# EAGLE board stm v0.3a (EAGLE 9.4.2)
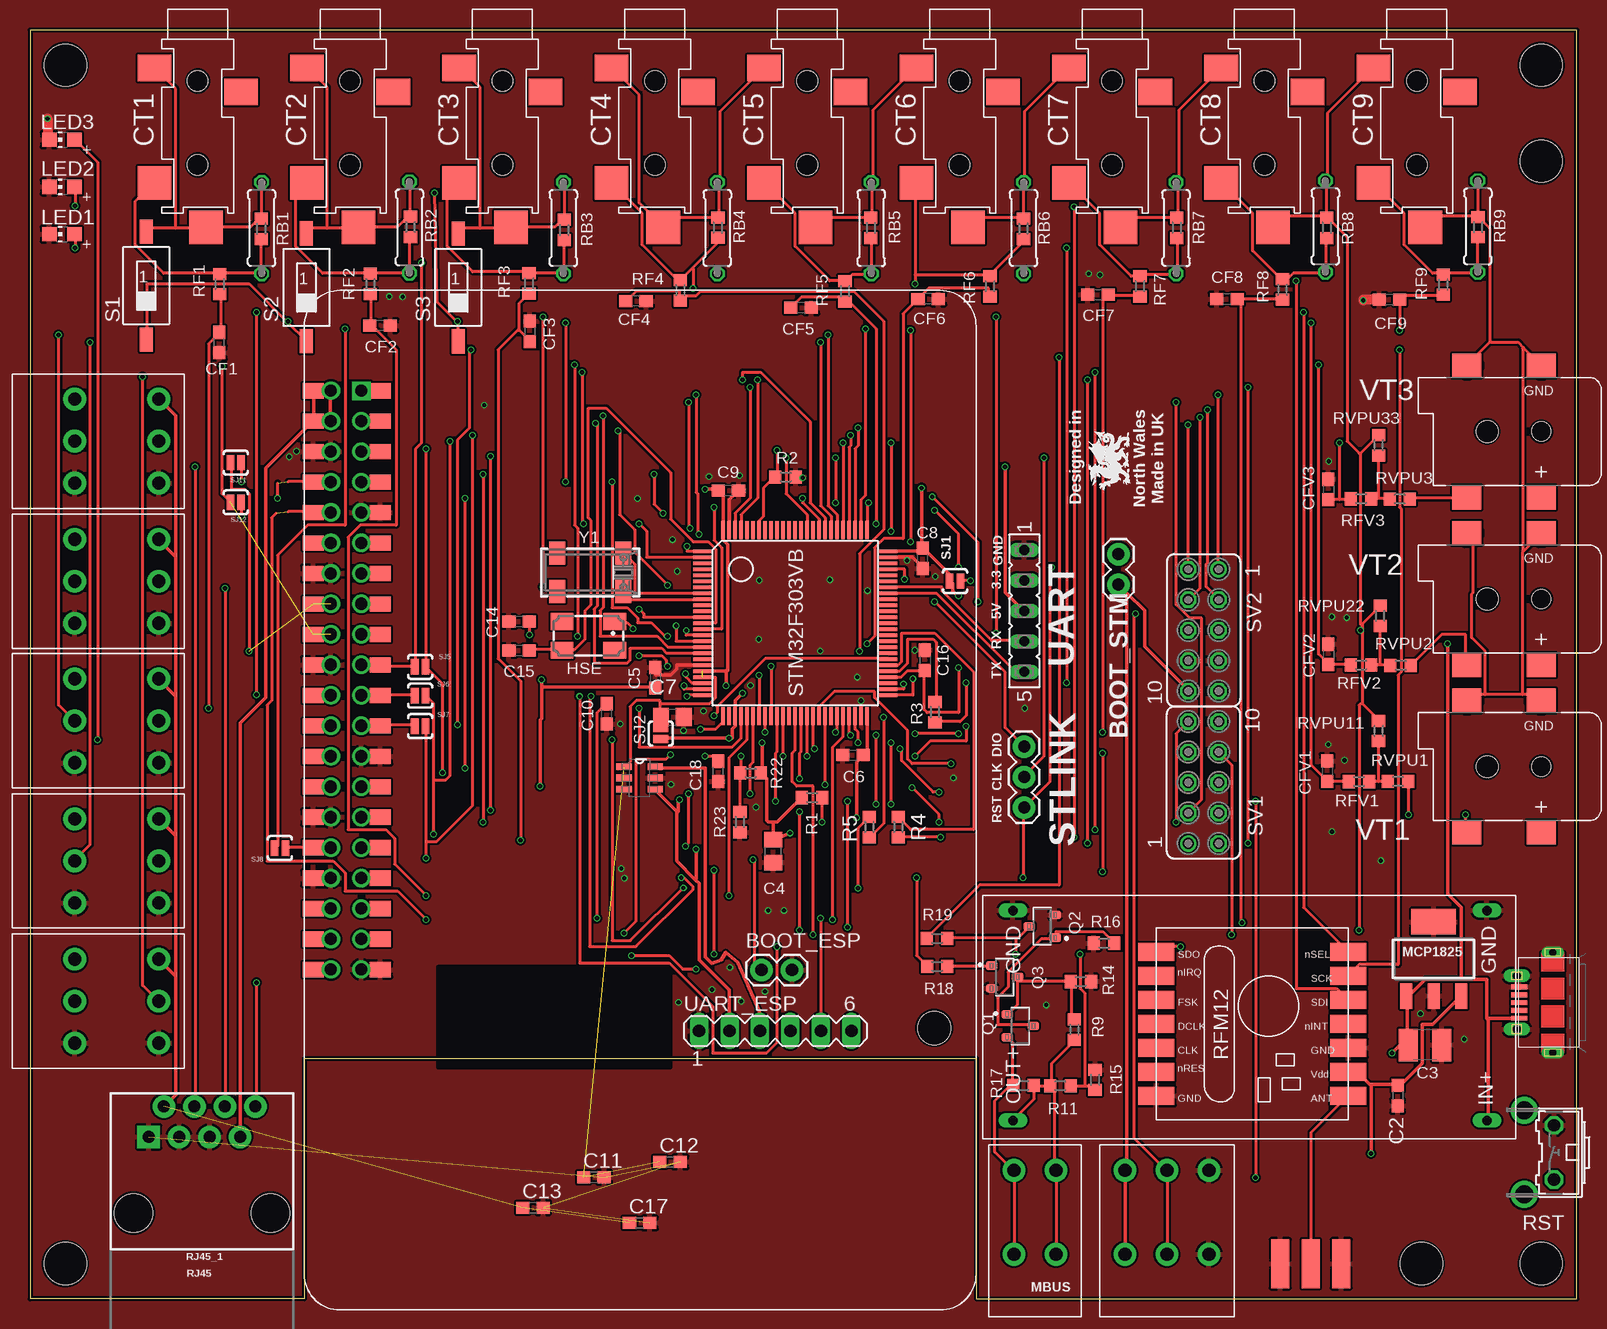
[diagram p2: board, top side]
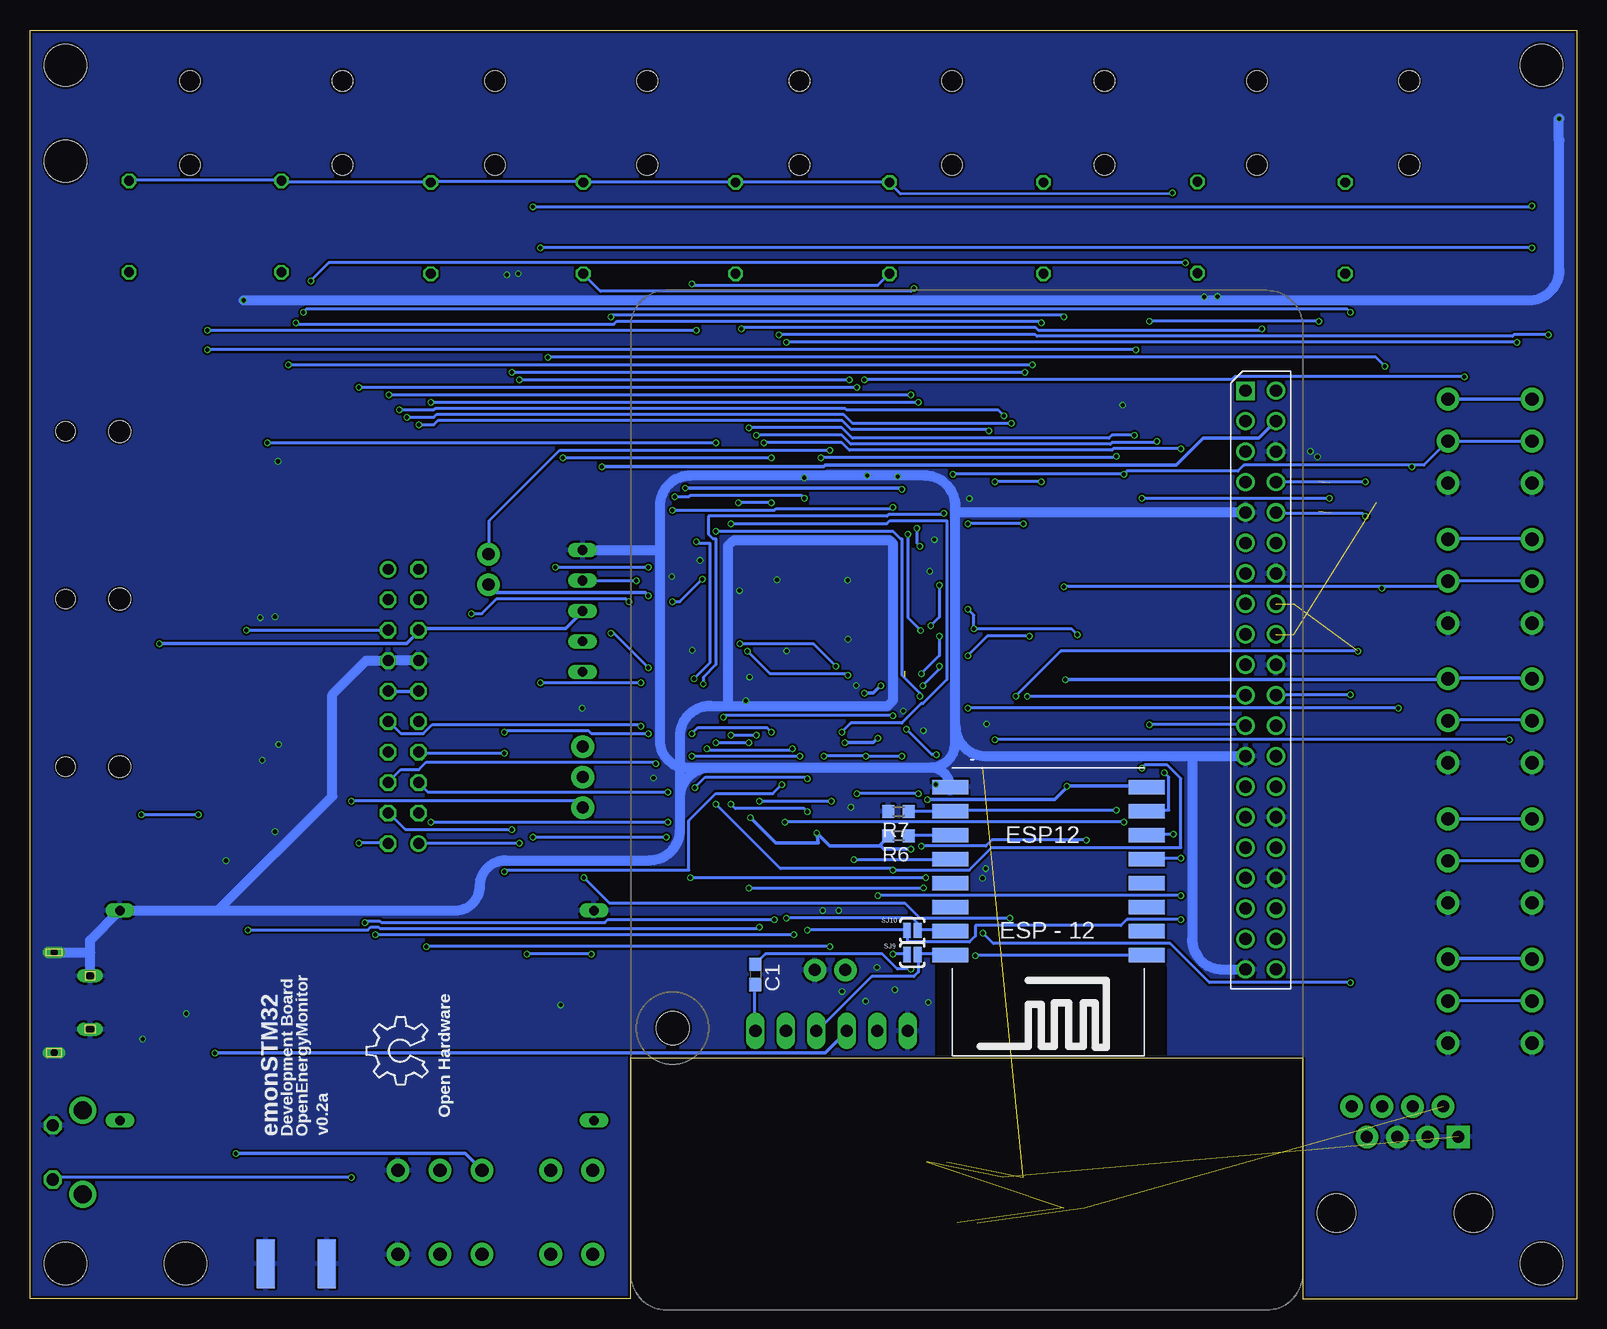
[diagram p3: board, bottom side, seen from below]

Size 128.91 x 105.79 mm. Coordinates in mm from the lower left corner, seen from the top.
Outline: 128.91,105.79 0,105.79 0,0 22.86,0 22.86,20.07 78.87,20.07 78.87,0 128.91,0 128.91,105.79
Copper layers (1*16): Top 0.035mm / dielectric 1.53mm / Bottom 0.035mm
Design rules "jlcpcb *": minimum track width 6mil, minimum drill 0.35mm, track to track 6mil, track to pad 6mil, pad to pad 7mil, via to via 8mil, smd to smd 0mil, copper to edge 8mil, drill to drill 10mil, minimum pad ring 3mil, minimum via ring 3mil, stop-mask expansion 2mil, vias tented up to drill 25mil, thermal gap 8mil
Net classes: 0 default: width 0.203 mm, drill 0.35 mm, clearance 0.152 mm; 1 power: width 0.279 mm, drill 0.35 mm, clearance 0.178 mm; 2 gnd: width 0.254 mm, drill 0.35 mm, clearance 0.152 mm
Holes 3.5 mm at 125.95,102.85 2.95,102.85 2.95,2.95 125.95,2.95 125.95,94.85 115.95,2.95
tRestrict: area 34,19.3 to 53.3,27.7
bRestrict: area 34.2,19.3 to 53.5,27.7

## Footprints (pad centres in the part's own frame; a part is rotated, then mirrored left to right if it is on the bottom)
OMNIMATE_LSF_2 = drill 1.1 pad 1.9: P$1 -3.5,-3.5; P$2 -3.5,3.5; P$3 0,-3.5; P$4 0,3.5
OMNIMATE_LSF_3 = drill 1.1 pad 1.9: P$1 -3.5,-3.5; P$2 -3.5,3.5; P$3 0,-3.5; P$4 0,3.5; P$5 3.5,-3.5; P$6 3.5,3.5
1X02 = drill 1.016 pad 1.88: 1 0,0; 2 2.54,0
C0603 = smd 1.1 x 1: 1 -0.85,0; 2 0.85,0
C1210 = smd 1.6 x 2.7: 1 -1.4,0; 2 1.4,0
C0805 = smd 1.3 x 1.5: 1 -0.95,0; 2 0.95,0
STEREO_SMT = smd 2.8 x 2.2: P$1 -3.6,-2.4; P$3 3.6,-4.4 | smd 2.8 x 2.8: P$2 -3.6,-12; P$4 0.7,-15.7 | hole 1.7: 0,-3.5; 0,-10.5
ESP12-SMD = smd 3 x 1.2: ADC -8.3,3.8; CH_PD -8.3,1.8; GND 8.1,-8.2; GPIO0 8.1,-2.2; GPIO2 8.1,-4.2; GPIO4 8.1,-0.2; GPIO5 8.1,1.8; GPIO12 -8.3,-4.2; GPIO13 -8.3,-6.2; GPIO14 -8.3,-2.2; GPIO15 8.1,-6.2; GPIO16 -8.3,-0.2; RESET -8.3,5.8; RXD0 8.1,3.8; TXD0 8.1,5.8; VCC -8.3,-8.2
FE05-1 = drill 0.813 long: 1 -5.08,0; 2 -2.54,0; 3 0,0; 4 2.54,0; 5 5.08,0
CTS406 = smd 1.9 x 1.4: 1 -2.2,-1.2; 2 2.2,-1.2; 3 2.2,1.2; 4 -2.2,1.2
SMA-EDGE = smd 1.524 x 4.064: GND@0 0,0; GND@1 5.08,0; SIG 2.54,0 | smd 1.524 x 4.064 bottom: GND@2 0,0; GND@3 5.08,0
CHIP-LED0805 = smd 1.2 x 1.2: A 0,-1.05; C 0,1.05
SOT-223 = smd 1 x 2.1: 1 -2.3,-3.1; 2 0,-3.1; 3 2.3,-3.1 | smd 3.7 x 2.1: 4 0,3.1
RPI3MIRROR2 = drill 1.016 square: P$1 8.37,4.775 | drill 1.016: P$2 8.357,2.233; P$3 10.897,4.773; P$4 10.897,2.233; P$5 13.437,4.773; P$6 13.437,2.233; P$7 15.977,4.773; P$8 15.977,2.233; P$9 18.517,4.773; P$10 18.517,2.233; P$11 21.057,4.773; P$12 21.057,2.233; P$13 23.597,4.773; P$14 23.597,2.233; P$15 26.137,4.773; P$16 26.137,2.233; P$17 28.677,4.773; P$18 28.677,2.233; P$19 31.217,4.773; P$20 31.217,2.233; P$21 33.757,4.773; P$22 33.757,2.233; P$23 36.297,4.773; P$24 36.297,2.233; P$25 38.837,4.773; P$26 38.837,2.233; P$27 41.377,4.773; P$28 41.377,2.233; P$29 43.917,4.773; P$30 43.917,2.233; P$31 46.457,4.773; P$32 46.457,2.233; P$33 48.997,4.773; P$34 48.997,2.233; P$35 51.537,4.773; P$36 51.537,2.233; P$37 54.077,4.773; P$38 54.077,2.233; P$39 56.617,4.773; P$40 56.617,2.233 | smd 1.27 x 1.778: P$41 8.371,6.351; P$42 8.371,0.763; P$43 10.911,6.351; P$44 10.911,0.763; P$45 13.451,6.351; P$46 13.451,0.763; P$47 15.991,6.351; P$48 15.991,0.763; P$49 18.531,6.351; P$50 18.531,0.763; P$51 21.071,6.351; P$52 21.071,0.763; P$53 23.611,6.351; P$54 23.611,0.763; P$55 26.151,6.351; P$56 26.151,0.763; P$57 28.691,6.351; P$58 28.691,0.763; P$59 31.231,6.351; P$60 31.231,0.763; P$61 33.771,6.351; P$62 33.771,0.763; P$63 36.311,6.351; P$64 36.311,0.763; P$65 38.851,6.351; P$66 38.851,0.763; P$67 41.391,6.351; P$68 41.391,0.763; P$69 43.931,6.351; P$70 43.931,0.763; P$71 46.471,6.351; P$72 46.471,0.763; P$73 49.011,6.351; P$74 49.011,0.763; P$75 51.551,6.351; P$76 51.551,0.763; P$77 54.091,6.351; P$78 54.091,0.763; P$79 56.631,6.351; P$80 56.631,0.763 | hole 2.75: 61.5,52.505
SOT23 = smd 0.71 x 0.96: 1 -0.95,-1.075; 2 0.95,-1.075; 3 0,1.075
R0603 = smd 1 x 1.1: 1 -0.85,0; 2 0.85,0
0207/7 = drill 0.813 octagon: 1 -3.81,0; 2 3.81,0
RFM12 = smd 1.5 x 3: 1 -5,-10; 2 -3,-10; 3 -1,-10; 4 1,-10; 5 3,-10; 6 5,-10; 7 7,-10; 8 7,6; 9 5,6; 10 3,6; 11 1,6; 12 -1,6; 13 -3,6; 14 -5,6
RJ45-8 = drill 1 pad 1.88 square: 1 -4.445,6.35 | drill 1 pad 1.88: 2 -3.175,8.89; 3 -1.905,6.35; 4 -0.635,8.89; 5 0.635,6.35; 6 1.905,8.89; 7 3.175,6.35; 8 4.445,8.89 | hole 3.2: -5.715,0; 5.715,0
B3F-31XX = drill 1.016 octagon: 1 -2.261,-1.245; 2 2.261,-1.245 | drill 1.499 pad 2.159: 3 -3.505,1.245; 4 3.505,1.245
SMS-001 = smd 1.092 x 2.007: 1 0,-4.496; 2 0,4.496
SJ_2S-NO = smd 0.635 x 1.27: 1 -0.45,0; 2 0.45,0
1X03 = drill 1.016 pad 1.88: 1 0,0; 2 2.54,0; 3 5.08,0
TQFP100 = smd 0.27 x 1.5: 1 -6,-7.75; 2 -5.5,-7.75; 3 -5,-7.75; 4 -4.5,-7.75; 5 -4,-7.75; 6 -3.5,-7.75; 7 -3,-7.75; 8 -2.5,-7.75; 9 -2,-7.75; 10 -1.5,-7.75; 11 -1,-7.75; 12 -0.5,-7.75; 13 0,-7.75; 14 0.5,-7.75; 15 1,-7.75; 16 1.5,-7.75; 17 2,-7.75; 18 2.5,-7.75; 19 3,-7.75; 20 3.5,-7.75; 21 4,-7.75; 22 4.5,-7.75; 23 5,-7.75; 24 5.5,-7.75; 25 6,-7.75; 51 6,7.75; 52 5.5,7.75; 53 5,7.75; 54 4.5,7.75; 55 4,7.75; 56 3.5,7.75; 57 3,7.75; 58 2.5,7.75; 59 2,7.75; 60 1.5,7.75; 61 1,7.75; 62 0.5,7.75; 63 0,7.75; 64 -0.5,7.75; 65 -1,7.75; 66 -1.5,7.75; 67 -2,7.75; 68 -2.5,7.75; 69 -3,7.75; 70 -3.5,7.75; 71 -4,7.75; 72 -4.5,7.75; 73 -5,7.75; 74 -5.5,7.75; 75 -6,7.75 | smd 1.5 x 0.27: 26 7.75,-6; 27 7.75,-5.5; 28 7.75,-5; 29 7.75,-4.5; 30 7.75,-4; 31 7.75,-3.5; 32 7.75,-3; 33 7.75,-2.5; 34 7.75,-2; 35 7.75,-1.5; 36 7.75,-1; 37 7.75,-0.5; 38 7.75,0; 39 7.75,0.5; 40 7.75,1; 41 7.75,1.5; 42 7.75,2; 43 7.75,2.5; 44 7.75,3; 45 7.75,3.5; 46 7.75,4; 47 7.75,4.5; 48 7.75,5; 49 7.75,5.5; 50 7.75,6; 76 -7.75,6; 77 -7.75,5.5; 78 -7.75,5; 79 -7.75,4.5; 80 -7.75,4; 81 -7.75,3.5; 82 -7.75,3; 83 -7.75,2.5; 84 -7.75,2; 85 -7.75,1.5; 86 -7.75,1; 87 -7.75,0.5; 88 -7.75,0; 89 -7.75,-0.5; 90 -7.75,-1; 91 -7.75,-1.5; 92 -7.75,-2; 93 -7.75,-2.5; 94 -7.75,-3; 95 -7.75,-3.5; 96 -7.75,-4; 97 -7.75,-4.5; 98 -7.75,-5; 99 -7.75,-5.5; 100 -7.75,-6
FE05-2 = drill 0.914: 1 -5.08,1.27 | drill 0.914 octagon: 2 -5.08,-1.27; 3 -2.54,1.27; 4 -2.54,-1.27; 5 0,1.27; 6 0,-1.27; 7 2.54,1.27; 8 2.54,-1.27; 9 5.08,1.27; 10 5.08,-1.27
47589-0001 = smd 1.35 x 0.4: 1 2.8,1.3; 2 2.8,0.65; 3 2.8,0; 4 2.8,-0.65; 5 2.8,-1.3 | drill 0.6 pad 0.95 long: CASING1 0,4.175; CASING2 0,-4.175 | drill 0.7 pad 1.1 long: CASING3 3,2.225; CASING4 3,-2.225
BOOST = drill 0.8 long: IN+ 17.5,39.5; OUT+ 17.5,0; P$1 0,0; P$2 0,39.5
SOT95P280X145-6N = smd 1.27 x 0.559: 1 -1.295,0.94; 2 -1.295,0; 3 -1.295,-0.94; 4 1.295,-0.94; 5 1.295,0; 6 1.295,0.94
MA06-1 = drill 1.016 long: 1 -6.35,0; 2 -3.81,0; 3 -1.27,0; 4 1.27,0; 5 3.81,0; 6 6.35,0
DCJACK_2MM_SMT = smd 2.4 x 2: GND 0,-5.5; GNDBREAK 6.2,-5.5; PWR1 0,5.5; PWR2 6.2,5.5 | hole 1.6: 0,0 | hole 1.8: 4.5,0
CRYSTAL_8X3.8 = smd 1.3 x 1.9: P$1 -2.75,-1.6; P$2 2.75,-1.6; P$3 2.75,1.6; P$4 -2.75,1.6

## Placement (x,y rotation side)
2POLE_MBUS  OMNIMATE_LSF_2  [OMNIMATE_LSF_2]  85.5,7.24 0 top
3POLE_1  OMNIMATE_LSF_3  [OMNIMATE_LSF_3]  7.23,71.51 270 top
3POLE_2  OMNIMATE_LSF_3  [OMNIMATE_LSF_3]  7.23,59.83 270 top
3POLE_3  OMNIMATE_LSF_3  [OMNIMATE_LSF_3]  7.23,48.2 270 top
3POLE_4  OMNIMATE_LSF_3  [OMNIMATE_LSF_3]  7.23,36.52 270 top
3POLE_5  OMNIMATE_LSF_3  [OMNIMATE_LSF_3]  7.23,24.83 270 top
3POLE_6  OMNIMATE_LSF_3  [OMNIMATE_LSF_3]  94.74,7.24 0 top
BOOT_ESP  [1X02]  60.96,27.43 0 top
BOOT_STM  [1X02]  90.7,62.09 270 top
C1  100nF  [C0603]  68.45,27.05 270 bottom
C2  100nF  [C0603]  113.97,16.96 270 top
C3  4.7uF  [C1210]  116.25,21.17 180 top
C4  4.7uF  [C0805]  61.93,37.33 90 top
C5  100nF  [C0603]  52.09,51.79 270 top
C6  100nF  [C0603]  68.59,45.34 0 top
C7  1uF  [C0805]  53.53,48.51 0 top
C8  100nF  [C0603]  74.39,61.75 90 top
C9  100nF  [C0603]  58.2,67.38 180 top
C10  100nF  [C0603]  48.08,48.78 90 top
C11  10nF  [C0603]  46.99,10.16 0 top
C12  1uF  [C0603]  53.34,11.43 0 top
C13  10nF  [C0603]  41.91,7.62 0 top
C14  18pF  [C0603]  40.76,56.47 180 top
C15  18pF  [C0603]  40.76,54.04 180 top
C16  100nF  [C0603]  74.58,53.24 270 top
C17  1uF  [C0603]  50.8,6.35 0 top
C18  10uF  [C0603]  57.36,43.98 90 top
CF1  100nF  [C0603]  15.79,79.74 90 top
CF2  100nF  [C0603]  29.17,81.16 180 top
CF3  100nF  [C0603]  41.63,80.66 270 top
CF4  100nF  [C0603]  50.49,83.19 180 top
CF5  100nF  [C0603]  64.25,82.64 180 top
CF6  100nF  [C0603]  74.84,83.37 180 top
CF7  100nF  [C0603]  89,83.73 0 top
CF8  100nF  [C0603]  99.74,83.37 0 top
CF9  100nF  [C0603]  113.3,83.33 0 top
CFV1  100nF  [C0603]  108.1,44 270 top
CFV2  100nF  [C0603]  108.2,53.74 270 top
CFV3  100nF  [C0603]  108.2,67.49 270 top
CT1  STEREO_SMD  [STEREO_SMT]  13.97,105.04 0 top
CT2  STEREO_SMD  [STEREO_SMT]  26.67,105.04 0 top
CT3  STEREO_SMD  [STEREO_SMT]  39.37,105.04 0 top
CT4  STEREO_SMD  [STEREO_SMT]  52.07,105.04 0 top
CT5  STEREO_SMD  [STEREO_SMT]  64.77,105.04 0 top
CT6  STEREO_SMD  [STEREO_SMT]  77.47,105.04 0 top
CT7  STEREO_SMD  [STEREO_SMT]  90.17,105.04 0 top
CT8  STEREO_SMD  [STEREO_SMT]  102.87,105.04 0 top
CT9  STEREO_SMD  [STEREO_SMT]  115.57,105.04 0 top
ESP12  [ESP12-SMD]  44.13,34.47 180 bottom
GND  UART  [FE05-1]  82.86,57.36 270 top
HSE  8MHZ  [CTS406]  46.54,55.29 180 top
J$1  SMA_EDGE  [SMA-EDGE]  104.18,2.93 0 top
LED1  Red 1.85V  [CHIP-LED0805]  2.67,88.77 90 top
LED2  Red 1.85V  [CHIP-LED0805]  2.67,92.71 90 top
LED3  Red 1.85V  [CHIP-LED0805]  2.67,96.65 90 top
LOGO1  OSHW_LOGO_6MILX0200-NT  [OSHW_6X200_NOTEXT]  95.78,17.86 90 bottom
MCP1825  MCP1825SOT-223-3  [SOT-223]  116.97,28.35 0 top
PCB2  RPI3YA  [RPI3MIRROR2]  22.84,84.09 270 top
Q1  MMBT3906  [SOT23]  82.52,22.77 270 top
Q2  MMBT3904  [SOT23]  84.34,31.07 90 top
Q3  MMBT3904  [SOT23]  81.21,26.85 270 top
R1  4.7k  [R0603]  65.18,41.79 180 top
R2  10k  [R0603]  62.97,68.51 0 top
R3  220R  [R0603]  75.41,48.93 90 top
R4  220R  [R0603]  72.36,39.34 90 top
R5  220R  [R0603]  69.95,39.34 270 top
R6  10k  [R0603]  56.52,38.61 180 bottom
R7  10k  [R0603]  56.52,40.64 180 bottom
R9  39K  [R0603]  87.03,22.46 270 top
R11  33K  [R0603]  85.86,17.77 180 top
R14  22K  [R0603]  87.57,26.46 180 top
R15  3k3  [R0603]  88.75,18.27 270 top
R16  82R  [R0603]  89.51,29.66 0 top
R17  220K  [R0603]  82.79,17.81 0 top
R18  1K  [R0603]  75.6,27.72 180 top
R19  1K  [R0603]  75.6,30.06 180 top
R22  10k  [R0603]  60.06,43.85 0 top
R23  10k  [R0603]  59.16,39.76 90 top
RB1  22r  [R0603]  19.27,89.22 90 top
RB2  22r  [R0603]  31.71,89.37 90 top
RB3  22r  [R0603]  44.52,89.12 90 top
RB4  22r  [R0603]  57.33,89.31 90 top
RB5  22r  [R0603]  70.07,89.29 90 top
RB6  22r  [R0603]  82.78,89.22 90 top
RB7  22r  [R0603]  95.56,89.3 90 top
RB8  22r  [R0603]  108.07,89.31 90 top
RB9  22r  [R0603]  120.67,89.36 90 top
RB10  22r  [0207/7]  19.3,89.28 90 top
RB11  22r  [0207/7]  31.62,89.33 90 top
RB12  22r  [0207/7]  44.45,89.28 90 top
RB13  22r  [0207/7]  57.28,89.28 90 top
RB14  22r  [0207/7]  70.1,89.28 90 top
RB15  22r  [0207/7]  82.8,89.28 90 top
RB16  22r  [0207/7]  95.5,89.28 90 top
RB17  22r  [0207/7]  107.95,89.41 90 top
RB18  22r  [0207/7]  120.65,89.41 90 top
RF1  330R  [R0603]  15.81,84.6 270 top
RF2  330R  [R0603]  28.36,84.62 270 top
RF3  330R  [R0603]  41.59,84.66 270 top
RF4  330R  [R0603]  54.2,84.09 270 top
RF5  330R  [R0603]  67.92,84.01 270 top
RF6  330R  [R0603]  80,84.41 270 top
RF7  330R  [R0603]  92.5,84.43 270 top
RF8  330R  [R0603]  104.38,84.16 270 top
RF9  330R  [R0603]  117.77,84.56 270 top
RFM69HCW  RFM12_SMDSMD  [RFM12]  103.86,23.92 270 top
RFV1  330R  [R0603]  110.75,43.13 180 top
RFV2  330R  [R0603]  110.93,52.85 180 top
RFV3  330R  [R0603]  110.92,66.72 180 top
RJ45_1  RJ45  [RJ45-8]  14.33,7.17 0 top
RST  [B3F-31XX]  125.76,12.21 90 top
RVPU1  120k  [R0603]  114,43.15 0 top
RVPU2  120k  [R0603]  114.22,52.82 0 top
RVPU3  120k  [R0603]  114.15,66.7 180 top
RVPU11  10k  [R0603]  112.38,47.36 90 top
RVPU22  10k  [R0603]  112.52,56.96 90 top
RVPU33  10k  [R0603]  112.39,71.18 90 top
S1  SWS001  [SMS-001]  9.69,84.49 180 top
S2  SWS001  [SMS-001]  23.04,84.34 180 top
S3  SWS001  [SMS-001]  35.69,84.33 180 top
SJ1  SOLDERJUMPERNO  [SJ_2S-NO]  77.09,59.85 180 top
SJ2  SOLDERJUMPERNO  [SJ_2S-NO]  52.56,47.13 90 top
SJ5  SOLDERJUMPERNO  [SJ_2S-NO]  32.51,52.7 180 top
SJ6  SOLDERJUMPERNO  [SJ_2S-NO]  32.51,50.29 180 top
SJ7  SOLDERJUMPERNO  [SJ_2S-NO]  32.51,47.75 180 top
SJ8  SOLDERJUMPERNO  [SJ_2S-NO]  20.83,37.59 180 top
SJ9  SOLDERJUMPERNO  [SJ_2S-NO]  55.37,28.7 0 bottom
SJ10  SOLDERJUMPERNO  [SJ_2S-NO]  55.37,30.73 180 bottom
SJ11  SOLDERJUMPERNO  [SJ_2S-NO]  17.14,69.72 180 top
SJ12  SOLDERJUMPERNO  [SJ_2S-NO]  17.14,66.42 180 top
STLINK  [1X03]  82.84,46.06 270 top
STM32F303VB  STM32F303XB  [TQFP100]  63.75,56.34 270 top
SV1  [FE05-2]  97.79,43.05 90 top
SV2  [FE05-2]  97.79,55.75 270 top
U$1  MICRO-USB-RECEPTACLE47589-0001  [47589-0001]  126.89,24.71 180 top
U$2  BOOST_MODULE  [BOOST]  81.92,32.38 270 top
U$8  MCP1501T-33E  [SOT95P280X145-6N]  50.8,43.43 0 top
UART_ESP  [MA06-1]  62.1,22.35 0 top
VT1  2.1MMJACKSMT  [DCJACK_2MM_SMT]  125.94,44.38 180 top
VT2  2.1MMJACKSMT  [DCJACK_2MM_SMT]  125.94,58.35 180 top
VT3  2.1MMJACKSMT  [DCJACK_2MM_SMT]  125.94,72.32 180 top
Y1  32.768kHz  [CRYSTAL_8X3.8]  46.69,60.58 180 top

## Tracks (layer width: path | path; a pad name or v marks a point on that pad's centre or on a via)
24V
  Top 0.254: R11.2 85,17.75 83.75,17.75 R17.2 83.62,17.75 83.62,16.62 82,15 U$2.OUT+ | R9.2 87,21.5 85.12,19.62 85.12,17.88 R11.2 | 2POLE_MBUS.P$3 85.5,10.62 2POLE_MBUS.P$4 85.38,10.75 85.38,17.75 85.25,17.88 R11.2
+3V3  (via drill 0.35)  (3 unrouted)
  Top 0.279: 111.75,17.88 111.62,17.88 110.62,18.88 109.88,18.88 RFM69HCW.9 | 111.75,17.88 113.88,17.88 C2.1 114,17.88 114.25,17.88 116,19.62 116,22.88 116.88,22.88 119.25,25.25 MCP1825.3 | 3POLE_6.P$1 91.25,10.62 3POLE_6.P$2 91.38,10.75 91.38,58.75 91.44,58.81 | C8.2 74.5,62.5 76.62,60.38 76.62,59.88 SJ1.2 76.75,59.75 76.88,59.62 76.88,59 77.25,58.62 v77.38,58.62 | STM32F303VB.75 71.53,62.35 74.38,62.35 74.38,62.5 C8.2 | 91.44,58.81 90.75,59.5 BOOT_STM.2 | 91.44,58.81 92.88,57.38 92.88,54.38 96.5,50.75 SV2.10 | v111.75,12.12 111.75,17.88 | 12.12,26.88 12.12,17 11.25,16.12 RJ45_1.2 | 12.12,26.88 10.75,28.25 3POLE_5.P$2 | 12.06,38.69 12.12,38.62 12.12,26.88 | 12.06,38.69 10.75,40 3POLE_4.P$2 | 12.06,50.31 12.12,50.25 12.12,38.75 12.06,38.69 | 12.06,50.31 10.75,51.62 3POLE_3.P$2 | 12.06,61.94 12.12,61.88 12.12,50.38 12.06,50.31 | 12.06,61.94 10.75,63.25 3POLE_2.P$2 | 3POLE_1.P$2 10.75,75 12.12,73.62 12.12,62 12.06,61.94 | 58.12,52.38 58,52.38 | 56.01,52.34 58,52.34 58,52.25 | 58.12,52.38 58.12,62.88 57.75,63.25 57.75,64 STM32F303VB.100 57.75,64.12 57.75,67 57.38,67.38 C9.2 57.25,67.5 v56.25,67.5 | SJ2.1 52.62,46.75 v58.25,46.75 58.5,46.75 58.5,47.5 58.75,47.75 58.75,48.5 STM32F303VB.28 58.75,48.62 58.75,49.88 v59.38,50.5 | STM32F303VB.50 69.75,48.5 69.75,45.62 69.5,45.38 C6.2 69.38,45.25 68.88,44.75 v68.88,40.12 | v63.34,38.84 62.76,38.62 62.27,38.62 C4.2 | R1.2 64.25,41.75 62.25,39.75 61.94,39.75 | C4.2 | v61,46.38 61,43.88 R22.2 61,43.75 61.38,43.38 61.38,39.88 61.5,39.75 61.94,39.75 | 42.62,51 52,51 C5.2 | 42.62,51 42.62,48.38 42.5,48.25 v42.5,42.75 | 53.88,40.62 52.12,42.38 U$8.4
  Top 0.279: 53.88,40.62 53.88,36.5 55.44,34.94 | 55.44,34.94 55.75,34.62 55.75,28.25 58.25,25.75 58.25,22.38 UART_ESP.2 | v54.12,41.62 54,41.5 54,40.62 53.88,40.62 | v55.5,37.5 55.5,35 55.44,34.94 | 42.62,51 v42.62,51.62 | v74.29,67.61 74.29,62.76 C8.2 | v58,51.12 58,52.25 | 58,52.25 58.12,52.38 | C4.2 61.93,39.74 61.94,39.75
  Bottom 0.279: SV2.10 96.62,50.62 99,50.62 SV2.9 | v77.38,58.62 77.62,58.88 90,58.88 90.62,59.5 BOOT_STM.2 | v111.75,12.12 92.62,12.12 3POLE_6.P$2 | 3POLE_1.P$1 3.75,75 10.62,75 3POLE_1.P$2 | 3POLE_2.P$1 3.75,63.38 10.62,63.38 3POLE_2.P$2 | 3POLE_3.P$1 3.75,51.75 10.62,51.75 3POLE_3.P$2 10.75,51.62 v42.62,51.62 | 3POLE_4.P$1 3.75,40 10.62,40 3POLE_4.P$2 | 3POLE_5.P$1 3.75,28.38 10.62,28.38 3POLE_5.P$2 | 57.38,38.5 58,37.88 58,37.75 | 57.38,38.5 57.26,38.62 | 57.38,38.5 R6.2 | v68.88,40.12 66.75,38 63.2,38 v63.34,38.84 62.24,37.75 58,37.75 | v58.25,46.75 58.62,46.38 v61,46.38 | v58,51.12 58.62,50.5 v59.38,50.5 | ESP12.VCC 35.88,42.75 v42.5,42.75 42.5,42.62 43.5,41.62 v54.12,41.62 | 58,37.75 57.75,37.5 v55.5,37.5 | v74.29,67.61 56.36,67.61 v56.25,67.5
+3V3_ADC  (3 unrouted)
  Top 0.203: C7.1 52.5,48.6 52.5,49.53
  Top 0.254: 52.5,49.66 52.5,49.53 52.5,47.62 SJ2.2 | 52.5,49.66 52.5,49.88 50.5,49.88 50,49.38 50,44.75 49.62,44.38 U$8.1 | 52.5,49.66 56.66,49.66 57.14,50.14 57.14,51.84 56.01,51.84
+5V  (via drill 0.35)
  Top 0.279: PCB2.P$4 25,73.25 25,75.5 PCB2.P$2 25,75.62 23.75,75.62 PCB2.P$42 23.62,75.62 23.62,73.25 PCB2.P$44 23.5,73.12 19.62,69.25 19.62,50.12 17.5,48 17.5,13.62 RJ45_1.7 | U$8.6 52.12,44.25 56.25,44.25 56.25,28.5 56.81,27.96 57.6,28.26 57.98,28.9 58.97,28.06 60.75,24 60.75,22.38 UART_ESP.3 | 121.5,23.38 124,23.38 U$1.1 | 121.5,23.38 121.5,15 U$2.IN+ | 119.25,26.62 121.38,26.62 121.38,23.38 121.5,23.38 | 119.25,26.62 116.25,26.62 114.88,25.25 MCP1825.1 114.75,25.25 114.75,21.25 C3.2 114.62,21.25 114.25,21.25 v113.5,20.5 | v118.12,54.62 118.12,33.75 119.25,32.62 119.25,26.62 | v81.25,69.38 81.25,58.88 82.75,57.38 GND.3
  Bottom 0.279: GND.3 82.88,57.25 84.25,55.88 96.5,55.88 SV2.6 96.5,55.62 97.5,54.62 v118.12,54.62 | v113.5,20.5 62.62,20.5 60.88,22.25 UART_ESP.3 | v81.25,69.38 62.75,69.38 62.62,69.5 33.38,69.5 31.12,71.75 26.5,71.75 25.12,73.12 PCB2.P$4
AC1  (via drill 0.35)
  Top 0.254: v114.88,40.38 114.88,43.12 RVPU1.2 | v119.62,40.38 119.62,39 VT1.PWR2
  Bottom 0.254: v119.62,40.38 v114.88,40.38
AC2
  Top 0.254: RVPU2.2 115.12,52.88 117.62,55.38 119.62,55.38 119.62,52.88 VT2.PWR2
AC3
  Top 0.254: RVPU3.1 115,66.75 119.62,66.75 VT3.PWR2
ADC0
  Top 0.254: 112.38,66.75 111.88,66.75 RFV3.1 | 112.38,66.75 113.25,66.75 RVPU3.2 | 112.38,66.75 112.38,70.25 RVPU33.1
ADC_RJ45IN  (via drill 0.35)
  Top 0.254: v55.88,47.5 57.13,47.5 57.73,48.1 STM32F303VB.26 | v53.38,45.38 53,45 50.5,45 50.5,31.5 v49.5,30.5 | v18.88,26.38 18.88,16.12 RJ45_1.8
  Bottom 0.254: v55.88,47.5 53.75,45.38 v53.38,45.38 | v49.5,30.5 48.62,29.62 33.88,29.62 30.62,26.38 v18.88,26.38
ANT
  Top 0.254: RFM69HCW.8 109.75,16.88 106.75,13.88 106.75,3 J$1.SIG
BIAS  (via drill 0.35)
  Top 0.254: 111,49.62 112.38,48.25 RVPU11.2 | 111,56.25 111,55.75 | 111,55.75 111,49.62 | 111,56.25 112.5,57.75 RVPU22.2 | 110.88,70.5 112.38,72 RVPU33.2 | 110.88,70.5 110.88,56.25 111,56.25 | v62.12,41.5 62.12,45.5 62.25,45.62 62.25,48.5 STM32F303VB.35 | v68.12,31 v68.12,41.5 | v110.75,30.75 110.75,49.5 110.88,49.62 111,49.62 | v110.88,55.75 111,55.75 | 124.38,50.38 125.88,50.38 125.88,50 VT1.GND | 124.38,50.38 121.25,50.38 | 121.25,50.38 120.12,50.38 119.75,50 VT1.GNDBREAK | 121.25,50.38 121.25,54 120.12,55.12 120.12,58.75 120.25,58.88 120.25,63.25 119.75,63.75 VT2.GNDBREAK | 124.44,62.31 124.38,62.25 124.38,50.38 | 124.44,62.31 125.88,63.75 VT2.GND | RB9.2 120.62,90.25 120.62,93.12 RB18.2 | 121.62,79.75 119.75,77.88 VT3.GNDBREAK | 121.62,79.75 121.62,89.25 120.75,90.12 RB9.2 | 124.44,79.31 124,79.75 121.62,79.75 | 124.44,79.31 125.88,77.88 VT3.GND | CT9.P$4 116.38,89.38 117.25,90.25 120.5,90.25 RB9.2 | 124.44,62.31 124.38,62.38 124.38,79.25 124.44,79.31 | CT7.P$4 90.88,89.38 91.62,90.12 95.5,90.12 RB7.2 95.62,90.25 95.62,93 RB16.2 95.75,93 95.75,99.12 99.25,102.62 CT8.P$1 | RB8.2 108,90.25 108,93.12 RB17.2 108.12,93.12 108.12,98.88 111.88,102.62 CT9.P$1 | CT8.P$4 103.62,89.38 104.5,90.25 107.88,90.25 RB8.2 | 21.44,81.44 18.25,84.62 9.75,84.62 9.75,80 S1.2 | 21.44,81.44 23,79.88 S2.2 | S3.2 35.62,79.88 v35.62,81.5 35.5,81.5 33.88,83.12 v33.71,92.2 | v21.5,81.5 21.44,81.44 | CT4.P$1 48.5,102.62 50.75,100.38 50.75,91.38 52.75,89.38 CT4.P$4 52.88,89.38 53.62,90.12 57.25,90.12 RB4.2 57.38,90.25 57.38,93 RB13.2 57.5,93 57.5,99 61.12,102.62 CT5.P$1 | CT5.P$4 65.5,89.38 66.25,90.12 70,90.12 RB5.2 70.12,90.25 70.12,93 RB14.2 70.25,93 70.25,99.12 73.75,102.62 CT6.P$1
  Top 0.254: CT6.P$4 78.25,89.38 79,90.12 82.62,90.12 RB6.2 82.75,90.12 82.75,93 RB15.2 82.88,93.12 82.88,99 86.5,102.62 CT7.P$1 | 110.88,70.5 110.75,70.5 109.75,71.5 109.75,88.5 108.12,90.12 RB8.2
  Bottom 0.254: v68.12,41.5 v62.12,41.5 | v68.12,31 68.25,30.88 99.75,30.88 99.88,31 100.5,31 100.75,30.75 v110.75,30.75 | v110.88,55.75 99.12,55.75 SV2.5 | v21.5,81.5 v35.62,81.5 | v33.71,92.2 56.38,92.12 57.25,93 RB13.2 57.38,93.12 70,93.12 RB14.2 70.12,93.12 82.75,93.12 RB15.2 82.88,93.12 95.5,93.12 RB16.2 95.62,93.12 107.88,93.12 RB17.2 108,93.25 120.62,93.25 RB18.2
BIAS_IN  (via drill 0.35)
  Top 0.254: R23.2 59.12,40.62 59.12,43.75 R22.1 59.25,43.88 v59.25,45.25 | v56.25,45.25 56.88,45.25 57.25,44.88 C18.2 | v62.75,45.25 62.75,48.5 STM32F303VB.36
  Bottom 0.254: v56.25,45.25 v59.25,45.25 v62.75,45.25
BIAS_SW1
  Top 0.254: RB10.2 19.25,93 19.25,90.12 RB1.2 19.12,90.12 18.38,89.38 14.75,89.38 CT1.P$4 14.62,89.25 12.12,89.25 | 12.12,89.25 10,89.25 9.75,89 S1.1 | 12.12,89.25 12.12,100.88 10.38,102.62 CT1.P$1
BIAS_SW2
  Top 0.254: RB11.2 31.62,93.12 31.62,90.25 RB2.2 31.5,90.25 30.62,89.38 27.38,89.38 CT2.P$4 27.25,89.25 24.75,89.25 | 24.75,89.25 23.5,89.25 23.12,88.88 S2.1 | 24.75,89.25 24.75,101 23.12,102.62 CT2.P$1
BIAS_SW3
  Top 0.254: RB12.2 44.5,93 44.5,90 RB3.2 44.38,90 43.75,89.38 40.12,89.38 CT3.P$4 40,89.25 37.5,89.25 | 37.5,89.25 36.12,89.25 35.75,88.88 S3.1 | 37.5,89.25 37.5,101 35.88,102.62 CT3.P$1
BOOT0  (via drill 0.35)
  Top 0.254: STM32F303VB.94 60.75,64.12 60.75,64.88 61.12,65.25 61.12,67.62 62,68.5 R2.1 62.25,68.5 v62.25,70.75
  Bottom 0.254: v62.25,70.75 84.75,70.75 90.62,64.88 90.62,62.12 BOOT_STM.1
CS_RFM69  (via drill 0.35)
  Top 0.254: PCB2.P$62 23.62,50.38 25,50.38 PCB2.P$22 | v106.12,82.25 106.12,32.62 109.75,29 RFM69HCW.14 | v18.88,50.38 v18.88,82.25
  Bottom 0.254: v106.12,82.25 105.88,82.5 19.12,82.5 v18.88,82.25 | v18.88,50.38 25,50.38 PCB2.P$22
CT1  (via drill 0.35)
  Top 0.254: RF1.2 15.88,83.75 15.88,80.62 CF1.2 15.75,80.5 14.88,79.62 v14.88,49.25 | v50.75,49.25 50.75,46 58.5,46 59.25,46.75 59.25,48.5 STM32F303VB.29
  Bottom 0.254: v14.88,49.25 v50.75,49.25
CT2  (via drill 0.35)
  Top 0.254: RF2.2 28.38,83.75 28.38,81.25 CF2.2 28.5,81.25 28.5,81.12 30.5,79.12 30.5,64.5 27.5,64.5 26.5,63.5 26.5,39.12 29.62,39.12 30.38,38.38 30.38,36.25 v33,33.62 | v58.25,33.62 58.25,45.12 59.75,46.62 59.75,48.5 STM32F303VB.30
  Bottom 0.254: v33,33.62 v58.25,33.62
CT3  (via drill 0.35)
  Top 0.254: 40.75,80.75 40.75,83 41.5,83.75 RF3.2 | 40.75,80.75 41.62,79.88 CF3.2 | v60,42.12 60,44.5 60.25,44.75 60.25,48.5 STM32F303VB.31 | v54.88,42.12 54.88,38 v54.62,37.75 | v40.88,38.25 40.88,51.5 39,53.38 39,79.12 40.62,80.75 40.75,80.75
  Bottom 0.254: v54.88,42.12 v60,42.12 | v54.62,37.75 49.25,37.75 48.75,38.25 v40.88,38.25
CT4  (via drill 0.35)
  Top 0.254: CF4.2 49.75,83.25 50.5,84 54.12,84 54.12,83.25 RF4.2 54.25,83.62 55.5,83.62 55.88,84 68.62,84 71.12,81.5 71.12,64.12 69.12,62.12 v69.12,54 | v60.75,52 60.75,48.62 STM32F303VB.32
  Bottom 0.254: v60.75,52 60.88,52.12 67.25,52.12 v69.12,54
CT5  (via drill 0.35)
  Top 0.254: CF5.2 63.5,82.75 64.25,83.5 67.88,83.5 67.88,83.25 RF5.2 68,83.38 70.5,80.88 v70.5,64.62 | v61.25,47.25 61.25,48.5 STM32F303VB.33
  Bottom 0.254: v61.25,47.25 60.5,48 56.25,48 54.62,49.62 54.5,49.62 52.5,51.62 52.5,64.88 57.25,64.88 57.5,64.62 v70.5,64.62
CT6  (via drill 0.35)
  Top 0.254: RF6.2 79.88,83.62 79.88,84.25 74.88,84.25 CF6.2 73.88,83.25 72.75,82.12 72.75,63.38 71.12,63.38 70.38,62.62 70.38,55.25 v69.75,54.62 | v61.75,52.75 61.75,48.62 STM32F303VB.34
  Bottom 0.254: v61.75,52.75 63.62,54.62 v69.75,54.62
CT7  (via drill 0.35)
  Top 0.254: RF7.2 92.5,83.62 89.88,83.62 CF7.2 89.75,83.62 89.38,83.25 v89.38,47.25 | v67.12,47.25 67.25,47.38 67.25,48.5 STM32F303VB.45 | v77.38,47.12 v73.75,47.12
  Bottom 0.254: v67.12,47.25 67.5,47.62 73.25,47.62 v73.75,47.12 | v77.38,47.12 82.12,47.12 82.38,47.38 89.25,47.38 v89.38,47.25
CT8  (via drill 0.35)
  Top 0.254: RF8.2 104.38,83.38 100.62,83.38 CF8.2 100.88,83.25 100.88,31.5 v101,31.38 | v66.88,31.62 66.88,46 67.75,46.88 67.75,48.5 STM32F303VB.46
  Bottom 0.254: v66.88,31.62 80.75,31.62 81,31.38 99.62,31.38 99.75,31.5 100.88,31.5 v101,31.38
CT9  (via drill 0.35)
  Top 0.254: RF9.2 117.75,83.62 114.5,83.62 114.25,83.38 CF9.2 114.12,83.25 v114.12,80.75 | STM32F303VB.51 73.57,50.34 v73.57,51.71 | v73.38,80.75 v73.38,63.12 | STM32F303VB.51
  Bottom 0.254: v73.57,51.71 72.25,53.03 72.25,63 73.25,63 v73.38,63.12 | v114.12,80.75 v73.38,80.75
DS18B20  (via drill 0.35)
  Top 0.254: v66,39.75 66,41.75 R1.1 | v37.75,68.75 v37.75,39.75 | v72.8,51.27 72.8,50.85 71.53,50.85 STM32F303VB.52 | v52.75,65.5 52,66.25 v52,68.75 | v13.75,69.38 13.75,16.12 RJ45_1.4
  Bottom 0.254: v37.75,39.75 v66,39.75 | 13.75,69.5 12.75,69.5 10.75,71.5 3POLE_1.P$4 10.62,71.5 3.75,71.5 3POLE_1.P$3 | 13.75,69.5 27.75,69.5 28.25,69 37.5,69 v37.75,68.75 v52,68.75 | v72.8,51.27 72.8,51.83 71.75,52.88 71.75,63.38 72,63.38 72.38,63.75 72.38,65.25 57.5,65.25 57.38,65.38 52.88,65.38 v52.75,65.5 | v13.75,69.38 13.75,69.5
GND  (via drill 0.35)  (4 unrouted)
  Top 0.279: STM32F303VB.20 53.88,52.85 53.88,52.5 53.38,52 52.12,52 52.12,52.62 C5.1 | v69.25,49.88 69.25,48.62 STM32F303VB.49 | 71.62,61.84 | STM32F303VB.74 71.62,61.84 | 71.62,61.84 73.53,61.84 74.38,61 C8.1 | STM32F303VB.99 58.25,64.12 58.25,66.62 59,67.38 C9.1 | v64.39,68.45 R2.2
  Top 0.813: CF9.1 111.18,83.33 arc90 v111.1,83.26 | v1.46,98.4 1.46,96.8 arc90 LED3.C
  Bottom 0.279: v69.25,49.88 69.25,49.46
  Bottom 0.813: U$1.CASING4 123.89,28.86 | 123.89,28.86 123.89,29.91 U$2.P$2 113.24,32.38 | 113.24,32.38 103.72,41.91 103.72,50.39 100.89,53.21 SV2.7 SV2.8 | 70.74,49.97 70.74,62.78 70.3,63.22 57.23,63.22 56.98,62.97 56.98,49.9 57.42,49.46 69.25,49.46 72.2,49.46 arc-90 74.74,46.92 74.74,41.77 | 113.24,32.38 93.46,32.38 arc-90 91.41,34.44 arc90 89.27,36.58 77.28,36.58 arc-90 74.74,39.12 74.74,41.77 | 74.74,41.77 arc90 72.2,44.31 | ESP12.GND arc-90 53.87,44.31 | 72.2,44.31 53.87,44.31 | 53.87,44.31 arc-90 51.79,46.39 51.79,47.79 | 76.42,62.43 76.42,66.1 arc90 73.88,68.64 54.33,68.64 arc90 51.79,66.1 51.79,65.56 | 76.42,62.43 76.42,46.53 arc-90 74.2,44.31 72.2,44.31 | 51.79,47.79 51.79,65.56 | 51.79,47.79 arc-90 49.25,45.25 32.07,45.25 | 32.07,45.25 PCB2.P$25 | PCB2.P$9 51.77,65.57 arc-90 51.79,65.56 | 32.07,45.25 32.07,30.01 arc-90 29.53,27.47 PCB2.P$39 | v111.1,83.26 3.99,83.26 arc-90 1.45,85.8 1.45,96.57 arc-90 1.53,96.65 1.53,98.33 arc90 v1.46,98.4 | GND.1 76.44,62.44 arc90 76.42,62.43 | U$1.CASING2 123.92,28.89 arc90 123.89,28.86
  other vias: 60.5,41 108.23,69.84 61.51,32.39 62.84,32.38 61.24,25.63 56.83,25.79 54.05,24.73 58.32,27.65 59.27,24.82 53.42,42.9 49.19,47.94 115.88,23.8 119.52,21.67 73.08,61.57 75.43,60.24 56.59,68.56 59.14,68.64 73.72,54.08 108.19,46.22 109.54,44.91 49.53,35.09 49.26,35.89 108.49,56.87 109.73,56.8 88.22,85.47 89.16,85.37 21.61,70.2 22.21,70.67 29.94,83.57 31.05,83.55 54.46,47.39 56.13,49.03 65.85,54.01 66.66,59.95 60.74,55 60.77,59.92 68.93,51.84 69.78,59.05 60.05,51.15 50.62,66.73 37.85,74.52 108.49,38.96 112.57,36.54 84.69,24.51 76.95,43.44 82.89,49.26 53.54,63.3 53.93,60.66
  pour Top (isolate 0.178): 139.22,-7.21 -8.73,-7.21 -8.73,108.6 139.22,108.6
  pour Bottom: -12.17,110.63 -12.17,-9.99 141.99,-9.99 141.99,110.63
HSE_IN  (via drill 0.35)
  Top 0.254: v41.62,55.38 41.62,56.38 C14.1 | v50.25,55.88 49.75,56.38 48.75,56.38 HSE.1 | STM32F303VB.12 55.99,56.83 51.12,56.83 51.12,57.12 v50.75,57.5
  Bottom 0.254: v41.62,55.38 42.12,55.88 v50.25,55.88 50.25,57 v50.75,57.5
HSE_OUT
  Top 0.254: C15.1 41.62,54.12 44.25,54.12 HSE.3 44.38,54.12 45.38,54.12 46.25,55 46.25,57.38 46.75,57.88 46.75,64.88 46.5,65.12 46.5,74.25 48,74.25 53.38,68.88 53.38,65 55.25,63.12 56.5,63.12 57.12,62.5 57.12,56.35 56.02,56.35 STM32F303VB.13
LED1
  Top 0.254: STM32F303VB.55 72.46,52.33 73.12,53 73.12,55 75.25,55 75.5,54.75 75.5,49.88 R3.2
LED2
  Top 0.254: STM32F303VB.56 71.53,52.82 72.32,52.82 72.62,53.12 72.62,55.5 75.38,55.5 78.62,52.25 78.62,39.12 73.38,39.12 72.38,40.12 R4.2
LED3  (via drill 0.35)
  Top 0.254: v71.12,48.5 71.12,39.62 70,38.5 R5.2 | v57,48.62 57.25,48.88 57.25,49.38 61.25,53.38 71.5,53.38 STM32F303VB.57
  Bottom 0.254: v71.12,48.5 71,48.62 v57,48.62
MBUS_RX  (via drill 0.35)  (2 unrouted)
  Top 0.254: v73.88,35.12 73.88,28.62 74.75,27.75 R18.2 | v54.26,35.13 54.47,35.13 55.25,34.36 55.25,34.13 50.49,29.38 46.62,29.38 46.62,50.12 v46.75,50.25 | v18.25,54 18.25,67.12 17.88,67.5 16.75,67.5 16.75,69.62 SJ11.2
  Bottom 0.254: v54.26,35.13 73.87,35.13 v73.88,35.12 | v46.75,50.25 43,54 v18.25,54
MBUS_TX  (via drill 0.35)  (2 unrouted)
  Top 0.254: v85.75,78.5 85.75,34.5 79.12,34.5 74.75,30.12 R19.2 | v16,77.75 16,67.12 16.62,66.5 SJ12.2
  Bottom 0.254: v85.75,78.5 16.75,78.5 v16,77.75
MISO  (via drill 0.35)
  Top 0.254: SJ6.2 32,50.38 29.25,50.38 PCB2.P$61 29.12,50.38 27.62,50.38 PCB2.P$21 | v95.88,29.38 94.25,29.38 93.88,29 RFM69HCW.1 | v62.25,29.38 62.25,21.38 61.38,20.5 56.88,20.5 56.88,24.38 53.25,28 45.8,28 v45.8,50.24
  Bottom 0.254: v62.25,29.38 v95.88,29.38 | v45.8,50.24 27.63,50.24 PCB2.P$21
MOSI  (via drill 0.35)
  Top 0.254: PCB2.P$19 27.62,52.88 29.12,52.88 PCB2.P$59 29.25,52.75 32,52.75 SJ5.2 32.12,52.75 32.12,70.88 32.62,71.38 v32.62,86.38 | v105.5,84.88 105.5,25.88 108.88,25.88 109.75,25 RFM69HCW.12
  Bottom 0.254: v105.5,84.88 104,86.38 v32.62,86.38
N$1  (via drill 0.35)
  Top 0.254: v78.38,59.88 77.62,59.88 SJ1.1
  Bottom 0.254: v78.38,59.88 82.75,59.88 GND.2
N$2
  Top 0.254: RB1.1 19.25,88.25 19.25,85.62 RB10.1 19.25,85.5 15.88,85.5 RF1.1 15.75,85.5 11.12,85.5 8.75,87.88 8.75,91.5 10.25,93 CT1.P$2
N$5  (via drill 0.35)
  Top 0.254: v75.88,38.5 72.38,38.5 R4.1 | v87,91.05 v87,38.5 | v3.75,91.12 3.75,92.62 LED2.A
  Bottom 0.254: v87,38.5 v75.88,38.5 | v3.75,91.12 3.82,91.05 v87,91.05
N$6  (via drill 0.35)
  Top 0.254: v69,34.25 69,39.25 69.88,40.12 R5.1 | v54.45,34.27 50.02,29.88 48.5,29.88 v48.5,46.62 | v5.62,46.62 5.62,94.75 3.75,96.62 LED3.A
  Bottom 0.254: v69,34.25 68.98,34.27 v54.45,34.27 | v5.62,46.62 v48.5,46.62
N$7  (via drill 0.35)
  Top 0.254: v60.25,36.62 60.38,36.5 60.38,28 60.88,27.5 BOOT_ESP.1
  Bottom 0.254: v60.25,36.62 52.25,36.62 ESP12.GPIO0
N$8
  Top 0.254: RB2.1 31.62,88.5 31.62,85.62 RB11.1 31.5,85.5 28.38,85.5 RF2.1 28.25,85.5 24.38,85.5 22.12,87.75 22.12,92.12 23,93 CT2.P$2
N$10
  Top 0.254: RB3.1 44.5,88.25 44.5,85.5 RB12.1 44.38,85.5 41.62,85.5 RF3.1 41.5,85.62 36.88,85.62 34.75,87.75 34.75,92 35.75,93 CT3.P$2
N$11
  Bottom 0.254: R6.1 55.62,38.62 52.25,38.62 ESP12.GPIO2
N$16
  Top 0.254: SJ8.1 21.38,37.62 23.5,37.62 PCB2.P$72 23.62,37.62 25,37.62 PCB2.P$32
N$22
  Top 0.254: PCB2.P$41 29.12,75.75 27.62,75.75 PCB2.P$1
N$24
  Top 0.254: PCB2.P$57 29.12,55.5 27.62,55.5 PCB2.P$17
N$29
  Top 0.254: Q1.2 81.5,21.75 81.88,21.38 81.88,17.88 R17.1 81.75,17.88 80.38,16.5 80.38,12.25 81.88,10.75 2POLE_MBUS.P$2 82,10.62 2POLE_MBUS.P$1
N$30
  Top 0.254: Q1.3 83.5,22.88 80.62,22.88 80.62,25.12 81.5,26 81.5,27.25 84.25,30 85.38,30 Q2.1 85.5,30.12 85.5,30.62 89.38,30.62 90.25,29.75 R16.2
N$31
  Top 0.254: R9.1 87,23.38 86.75,23.62 86.75,26.38 R14.2 86.62,26.5 82.38,26.5 Q3.3 82.25,26.75 82.25,24.5 81.5,23.75 Q1.1
N$32  (via drill 0.35)
  Top 0.254: 87.88,17.75 86.75,17.75 R11.1 | 87.88,17.75 88.5,17.75 88.75,17.5 R15.2 | 82.12,30.12 76.5,30.12 R19.1 | 82.12,30.12 82.38,30.12 83.25,31 Q2.3 | 87.88,17.75 87.88,25.5 87.5,25.88 v87.5,28.75 | 82.12,30.12 v82.12,28.75
  Bottom 0.254: v82.12,28.75 v87.5,28.75
N$33
  Top 0.254: Q3.1 80.12,27.75 76.5,27.75 R18.1
N$34
  Top 0.254: 112.5,52.88 111.88,52.88 RFV2.1 | 112.5,52.88 113.25,52.88 RVPU2.1 | 112.5,52.88 112.5,56 RVPU22.1
N$37
  Top 0.254: 112.38,43.12 113.12,43.12 RVPU1.1 | 112.38,43.12 111.62,43.12 RFV1.1 | 112.38,43.12 RVPU11.1
N$38  (via drill 0.35)
  Top 0.254: 55.19,85.94 57.25,88 57.25,88.38 RB4.1 | 55.19,85.94 54.25,85 RF4.1 54.12,85 53.88,85 51,87.88 51,90.5 48.5,93 CT4.P$2 | v55.25,84.25 55.25,85.88 55.19,85.94
  Bottom 0.254: v55.25,84.25 55.5,84 81.38,84 82.75,85.38 RB15.1
N$39
  Top 0.254: RB5.1 70.12,88.38 70.12,85.5 RB14.1 70,85.38 68.5,85.38 68,84.88 RF5.1 67.88,84.88 66.62,84.88 63.75,87.75 63.75,90.5 61.25,93 CT5.P$2
N$40  (via drill 0.35)
  Top 0.254: RB6.1 82.75,88.25 82.75,88.12 80,85.38 RF6.1 79.88,85.38 73.75,85.38 | 73.75,85.38 73.75,93 CT6.P$2 | 73.75,85.38 v73.75,84.62
  Bottom 0.254: v73.75,84.62 73.62,84.5 58.25,84.5 57.38,85.38 RB13.1
N$41  (via drill 0.35)
  Top 0.254: v78,51.38 78,48.62 77.5,48.12 75.5,48.12 R3.1 | v86.38,87.62 v86.38,51.38 | v3.75,87.62 3.75,88.75 LED1.A
  Bottom 0.254: v86.38,51.38 v78,51.38 | v3.75,87.62 v86.38,87.62
N$42
  Top 0.254: RB7.1 95.62,88.38 95.62,85.5 RB16.1 95.5,85.38 92.62,85.38 RF7.1 92.38,85.25 91.75,85.25 89.12,87.88 89.12,90.5 86.62,93 CT7.P$2
N$43
  Top 0.254: RB8.1 108,88.38 108,85.62 RB17.1 107.88,85.5 105.25,85.5 104.88,85.12 104.5,85.12 RF8.1 104.25,85 101.88,87.38 101.88,90.5 99.38,93 CT8.P$2
N$44
  Top 0.254: RB9.1 120.62,88.5 120.62,85.62 RB18.1 120.62,85.5 117.88,85.5 RF9.1 117.75,85.5 116.88,85.5 114.5,87.88 114.5,90.5 112,93 CT9.P$2
NRST  (via drill 0.35)
  Top 0.254: v47.25,31.75 47.25,48.88 48,49.62 C10.2 | v82.75,35.12 82.75,40.88 STLINK.3 82.88,41 85,43.12 85,60.88 v85.12,61 | v57,66 57,63.25 57.62,62.62 57.62,55.84 STM32F303VB.14 | v75.38,65.75 77.38,63.75 v77.38,61 | v102.12,41.5 v102.12,10.12
  Bottom 0.254: v47.25,31.75 54.75,31.75 56,33 80.62,33 v82.75,35.12 | v57,66 57.12,65.88 66.75,65.88 66.88,65.75 v75.38,65.75 | v85.12,61 v77.38,61 | v102.12,10.12 126.88,10.12 127,10 RST.1 | v102.12,41.5 83.38,41.5 82.88,41 STLINK.3
PC0  (via drill 0.35)
  Top 0.254: STM32F303VB.15 54.69,55.33 v54.69,55.73 | v55.75,63.75 55.62,63.88 55.62,67.12 55.5,67.25 v55.5,75.38 | v99,75.38 99,60.88 SV2.1
  Bottom 0.254: v54.69,55.73 55.75,56.79 v55.75,63.75 | v99,75.38 v55.5,75.38
PC1  (via drill 0.35)
  Top 0.254: v53.84,56.13 53.84,54.84 STM32F303VB.16 | v53.12,59.5 50.38,62.25 50.38,64.12 49.12,65.38 49.12,72.25 v49,72.38 | v96.5,72.88 96.5,60.88 SV2.2
  Bottom 0.254: v53.84,56.13 53.12,56.85 v53.12,59.5 | v49,72.38 49.12,72.5 60.5,72.5 61.25,73.25 94.88,73.25 95.25,72.88 v96.5,72.88
PC2  (via drill 0.35)
  Top 0.254: STM32F303VB.17 53.17,54.33 52.25,55.25 47.5,55.25 47.5,57.38 47.75,57.62 v47.75,73.62 | v98.12,74.12 98.12,61.38 98,61.25 98,59.38 99,58.38 SV2.3
  Bottom 0.254: v47.75,73.62 48.25,74.12 60.88,74.12 61,74.25 95.12,74.25 95.25,74.12 v98.12,74.12
PC3  (via drill 0.35)
  Top 0.254: STM32F303VB.18 53.04,53.83 52.62,54.25 50,54.25 50,53.25 49.75,53 47,53 47,57.5 47.25,57.75 47.25,72.88 v47.12,73 | v97.5,73.5 97.5,59.25 96.62,58.38 SV2.4
  Bottom 0.254: v47.12,73 60.38,73 61.12,73.75 95,73.75 95.25,73.5 v97.5,73.5
PC14
  Top 0.254: STM32F303VB.8 55.97,58.84 50.38,58.84 50.38,61.25 49.5,62.12 Y1.P$1
PC15
  Top 0.254: STM32F303VB.9 55.99,58.33 49.5,58.33 49.5,58.88 Y1.P$4
PE0  (via drill 0.35)
  Top 0.254: v60.62,76.62 60.62,66.75 59.25,65.38 59.25,64.12 STM32F303VB.97 | v88.12,38 v88.12,76.62
  Bottom 0.254: v88.12,76.62 v60.62,76.62 | v88.12,38 96.5,38 SV1.1
PE1  (via drill 0.35)
  Top 0.254: v60,76 60,66.75 58.75,65.5 58.75,64.12 STM32F303VB.98 | v101.5,38 v101.5,76
  Bottom 0.254: v101.5,76 v60,76 | v101.5,38 99.12,38 SV1.2
PE2  (via drill 0.35)
  Top 0.254: v54.75,62.75 54.75,62.34 STM32F303VB.1 | v55,64.25 54.88,64.38 v54.88,74.75 | v95.5,74.75 95.5,57.88 96.62,56.75 97.62,56.75 97.62,41.62 96.62,40.62 SV1.3
  Bottom 0.254: v54.75,62.75 55,63 v55,64.25 | v95.5,74.75 v54.88,74.75
PE3  (via drill 0.35)
  Top 0.254: v50.75,64.62 51.38,64 51.38,61.85 STM32F303VB.2 | v46.12,64.62 46,64.75 v46,77.25 | v88.75,39.12 v88.75,77.25
  Bottom 0.254: v46.12,64.62 v50.75,64.62 | v88.75,77.25 v46,77.25 | v88.75,39.12 97.62,39.12 99,40.5 SV1.4
PE7  (via drill 0.35)
  Top 0.254: v65.25,30.38 65.25,42.75 63.88,42.75 63.5,43.12 63.5,45.5 63.75,45.75 63.75,48.5 STM32F303VB.38 | v100.12,30.38 100.12,44.5 99.12,45.5 SV1.8
  Bottom 0.254: v100.12,30.38 v65.25,30.38
PE8  (via drill 0.35)
  Top 0.254: v64.12,43.38 64.12,45.5 64.25,45.62 64.25,48.5 STM32F303VB.39 | v73.5,42.62 75.75,40.38 v75.75,39.75 | v95.5,39.75 95.5,47.12 96.5,48.12 SV1.9
  Bottom 0.254: v64.12,43.38 64.25,43.5 72.62,43.5 v73.5,42.62 | v95.5,39.75 v75.75,39.75
PE9  (via drill 0.35)
  Top 0.254: v64.75,45.25 64.75,48.5 STM32F303VB.40 | v73.75,45.25 75,46.5 78,46.5 v78,47.75
  Bottom 0.254: v73.75,45.25 v64.75,45.25 | v78,47.75 78.12,47.88 95.38,47.88 96.12,47.12 98,47.12 99,48.12 SV1.10
PE10  (via drill 0.35)
  Top 0.254: v65.38,45.88 65.25,46 65.25,48.5 STM32F303VB.41 | v72.5,45.88 72.62,45.75 72.62,44.88 75.25,42.25 v75.75,42.25
  Bottom 0.254: v65.38,45.88 65.5,45.75 72.38,45.75 v72.5,45.88 | v75.75,42.25 95.75,42.25 96.5,43 SV1.5
PE11  (via drill 0.35)
  Top 0.254: v76.75,44.62 73.5,44.62 73.12,45 73.12,47.38 70.38,50.12 70.38,50.62 67,50.62 65.75,49.38 65.75,48.62 STM32F303VB.42
  Bottom 0.254: v76.75,44.62 76.88,44.75 95.88,44.75 96.5,44.12 98,44.12 99,43.12 SV1.6
PE12  (via drill 0.35)
  Top 0.254: v66.25,42.88 66.25,48.5 STM32F303VB.43 | v89.38,45.5 v89.38,35.62
  Bottom 0.254: v66.25,42.88 67,42.12 71.75,42.12 74,39.88 74,35.75 89.25,35.75 v89.38,35.62 | v89.38,45.5 96.5,45.5 SV1.7
PULSE  (via drill 0.35)
  Top 0.254: STM32F303VB.54 72.58,51.83 73.12,52.38 74.5,52.38 C16.2 74.5,52.25 74.5,49.12 74.75,48.88 77.38,48.88 v77.38,52.62 | v80.5,81.88 v80.5,55.5 | v42.75,59.38 v42.75,81.88 | v16.25,59.25 16.25,16.12 RJ45_1.6
  Bottom 0.254: v77.38,52.62 80.25,55.5 v80.5,55.5 | v80.5,81.88 80.38,82 42.88,82 v42.75,81.88 | 16.25,59.38 11.12,59.38 10.75,59.75 3POLE_2.P$4 10.62,59.88 3.75,59.88 3POLE_2.P$3 | 16.25,59.38 v42.75,59.38 | v16.25,59.25 16.25,59.38
PUSHIN_3  (via drill 0.35)
  Top 0.254: v66.5,80.38 66.5,66.12 67.25,65.38 67.25,64.12 STM32F303VB.81 | v2.38,80.38 2.38,49.5 3.62,48.25 3POLE_3.P$3
  Bottom 0.254: v66.5,80.38 45.12,80.38 45,80.25 5.38,80.25 5.25,80.38 v2.38,80.38 | 3POLE_3.P$4 10.62,48.25 3.75,48.25 3POLE_3.P$3
PUSHIN_4  (via drill 0.35)
  Top 0.254: v65.88,79.75 65.88,66.12 66.75,65.25 66.75,64.12 STM32F303VB.82 | v5,79.75 5,37.88 3.75,36.62 3POLE_4.P$3
  Bottom 0.254: v5,79.75 v65.88,79.75 | 3POLE_4.P$4 10.62,36.5 3.75,36.5 3POLE_4.P$3
PUSHIN_5  (via drill 0.35)
  Top 0.254: v59.38,76.62 59.38,77.25 60.88,77.25 65,73.12 65,66.38 66.25,65.12 66.25,64.12 STM32F303VB.83 | v9.38,76.88 9.38,26.12 10.62,24.88 3POLE_5.P$4
  Bottom 0.254: v59.38,76.62 28.75,76.62 28.5,76.88 v9.38,76.88 | 3POLE_5.P$3 3.75,24.88 10.62,24.88 3POLE_5.P$4
PUSHIN_6  (via drill 0.35)
  Top 0.254: v64.38,66.75 64.38,66.38 65.75,65 65.75,64.12 STM32F303VB.84 | v75.18,66.88 79,63.06 v79,58.12 | v92.12,57.12 92,57 92,13.38 94.62,10.75 3POLE_6.P$4 94.75,10.62 3POLE_6.P$3
  Bottom 0.254: v64.38,66.75 64.62,67 73.88,67 73.99,66.88 v75.18,66.88 | v79,58.12 79.25,58.38 90,58.38 91.25,57.12 v92.12,57.12
RST_ESP_1
  Bottom 0.254: C1.2 68.5,26.12 68.5,22.38 UART_ESP.6
RST_ESP_2  (via drill 0.35)
  Top 0.254: v55.5,27.5 54.38,27.5 53.25,28.62 v50.12,28.62
  Bottom 0.254: v55.5,27.5 56.62,27.5 57.88,28.75 67.62,28.75 68.38,28 C1.1 | v50.12,28.62 35.88,28.62 ESP12.RESET
SPI3_CLK  (via drill 0.35)
  Top 0.254: v33,36.75 33,38.12 | 33,38.12 33,47.75 SJ7.1 | v69,72.62 69,71.12 68.75,70.88 68.75,64.12 STM32F303VB.78 | v36.88,72 36.88,41.12 33.88,38.12 33,38.12
  Bottom 0.254: v33,36.75 35.75,36.75 ESP12.GPIO14 | v69,72.62 61.25,72.62 60.38,71.75 39,71.75 38.75,72 v36.88,72
SPI3_CS  (via drill 0.35)
  Top 0.254: v26.25,80.88 26.25,64.5 23.12,64.5 20.62,62 20.62,37.75 20.5,37.62 SJ8.2 | v69.62,80.88 69.62,67 69.25,66.62 69.25,64.12 STM32F303VB.77
  Bottom 0.254: v26.25,80.88 26.38,80.75 44.88,80.75 45.12,81 69.5,81 v69.62,80.88
SPI3_CS_ESP  (via drill 0.35)
  Top 0.254: v63,70.12 63,67.12 64.75,65.38 64.75,64.12 STM32F303VB.86 | v38.38,40.75 v38.38,70.25
  Bottom 0.254: R7.1 55.62,40.62 52.25,40.62 ESP12.GPIO15 52.12,40.75 v38.38,40.75 | v63,70.12 38.5,70.12 v38.38,70.25
SPI3_MISO  (via drill 0.35)
  Top 0.254: v33.62,38.75 33.62,43.25 | 33.62,43.25 33.62,49.62 33,50.25 SJ6.1 | v68.38,72 68.38,71.12 68.25,71 68.25,64.12 STM32F303VB.79 | v35,71.5 35,43.62 34.62,43.25 33.62,43.25
  Bottom 0.254: v33.62,38.75 35.75,38.75 ESP12.GPIO12 | v68.38,72 61.25,72 60.5,71.25 38.88,71.25 38.75,71.38 35.12,71.38 v35,71.5
SPI3_MOSI  (via drill 0.35)
  Top 0.254: v34.38,43.88 34.38,51.25 33,52.62 SJ5.1 33,52.75 v33,70.88 | v67.75,71.38 67.75,64.12 STM32F303VB.80
  Bottom 0.254: v34.38,43.88 34,43.5 34,40.75 35.75,40.75 ESP12.GPIO13 | v67.75,71.38 61.25,71.38 60.62,70.75 38.75,70.75 38.62,70.88 v33,70.88
SPI_CLK  (via drill 0.35)
  Top 0.254: SJ7.2 32,47.88 29.25,47.88 PCB2.P$63 29.12,47.88 27.62,47.88 PCB2.P$23 | v114.12,79.12 114.12,66 114.25,65.88 114.25,52.25 114,52 114,27.88 110.75,27.88 109.88,27 RFM69HCW.13 | v36.75,79.12 36.62,79 36.62,72.62 35.62,71.62 v35.62,47.88
  Bottom 0.254: v36.75,79.12 v114.12,79.12 | v35.62,47.88 27.62,47.88 PCB2.P$23
SWCLK  (via drill 0.35)
  Top 0.254: v69.88,66.38 69.76,66.26 69.76,64.09 STM32F303VB.76 | v67.12,70.12 v67.12,66.38 | v84.5,70.12 84.5,45.25 82.88,43.62 STLINK.2
  Bottom 0.254: v67.12,66.38 v69.88,66.38 | v84.5,70.12 v67.12,70.12
SWDIO  (via drill 0.35)
  Top 0.254: STM32F303VB.72 72.88,60.84 v72.88,60 | v75.38,58.12 81.25,52.25 81.25,47.62 82.75,46.12 STLINK.1 | STM32F303VB.72
  Bottom 0.254: v72.88,60 74.75,58.12 v75.38,58.12
UART_RX
  Top 0.254: STM32F303VB.69 76,59.34 76,59 80.12,54.88 82.75,54.88 GND.4 | STM32F303VB.69
UART_RX_ESP
  Bottom 0.254: ESP12.TXD0 52.25,28.75 54.88,28.75 SJ9.2 54.88,28.62 54.88,27.25 55.25,26.88 58.75,26.88 63.25,22.38 UART_ESP.4
UART_TX
  Top 0.254: STM32F303VB.68 71.52,58.83 75.55,58.83 82,52.38 82.75,52.38 GND.5
UART_TX_ESP  (via drill 0.35)
  Top 0.254: v65.88,31.75 65.88,22.38 UART_ESP.5
  Bottom 0.254: ESP12.RXD0 52.25,30.75 54.88,30.75 SJ10.1 54.88,30.88 54.88,31.25 55.38,31.75 v65.88,31.75
USART3_RX  (via drill 0.35)  (1 unrouted)
  Top 0.254: v20.62,66.75 20.62,68 | v36.25,44.25 v36.25,66.75 | v57,28.75 v57,35.75 | v69,46.38 69,47.25 68.75,47.5 68.75,48.5 STM32F303VB.48 | v71.75,41.25 v71.75,46.38 | 21.5,68.12 23.5,68.12 PCB2.P$48 23.62,68.12 25,68.12 PCB2.P$8 | v17.62,68.12 17.62,69.62 SJ11.1
  Bottom 0.254: v36.25,66.75 v20.62,66.75 | v36.25,44.25 36,44.5 34.12,44.5 33,43.38 33,37.62 48.75,37.62 50.62,35.75 v57,35.75 57,35.88 66.38,35.88 v71.75,41.25 | v57,28.75 55.88,28.75 SJ9.1 | v71.75,46.38 v69,46.38 | v17.62,68.12 25,68.12 PCB2.P$8
USART3_TX  (via drill 0.35)  (1 unrouted)
  Top 0.254: v33,31.62 30.62,34 26.25,34 26.25,35.5 25.25,36.5 19.75,36.5 19.75,49.5 20.12,49.88 20.12,65.12 20.5,65.5 | v68.38,47 68.25,47.12 68.25,48.5 STM32F303VB.47 | v70.5,41.25 v70.5,47 | v64.12,30.75 v64.12,40.62 | 21.5,65.62 23.5,65.62 PCB2.P$50 23.62,65.62 25,65.62 PCB2.P$10 | v17.62,65.25 17.62,66.38 SJ12.1
  Bottom 0.254: v33,31.62 37.5,31.62 38,31.12 50.12,31.12 50.12,30.25 50.62,29.75 55.75,29.75 55.75,30.62 SJ10.2 55.88,30.75 v64.12,30.75 | v70.5,47 v68.38,47 | v70.5,41.25 70.12,40.88 64.38,40.88 v64.12,40.62 | v17.62,65.25 17.88,65.5 25,65.5 PCB2.P$10
VSIG1  (via drill 0.35)
  Top 0.254: RFV1.2 109.88,43.12 108.12,43.12 CFV1.2 108,43.25 106.75,44.5 v106.75,81.38 | STM32F303VB.23 55.16,51.34 54.62,51.88 v54.62,52.12 | v53.12,55.25 52.88,55.25 51.75,56.38 50.62,56.38 50.62,56.75 49.75,57.62 48.5,57.62 v48.5,68.12 | v44.62,81.38 v44.62,68.12
  Bottom 0.254: v54.62,52.12 53.12,53.62 v53.12,55.25 | v44.62,68.12 v48.5,68.12 | v44.62,81.38 44.75,81.5 80,81.5 80.25,81.25 106.62,81.25 v106.75,81.38
VSIG2  (via drill 0.35)
  Top 0.254: RFV2.2 110,52.88 108.25,52.88 CFV2.2 108.12,53 107.38,53.75 v107.38,77.88 | STM32F303VB.24 54.5,50.83 v54.5,51.12 | v53.12,52.75 53,52.88 53,53.25 52.62,53.62 v50.75,53.62 | v45.62,55.25 45.62,64.25 45.38,64.5 v45.38,77.88
  Bottom 0.254: v54.5,51.12 53.12,52.5 v53.12,52.75 | v50.75,53.62 49.12,55.25 v45.62,55.25 | v107.38,77.88 v45.38,77.88
VSIG3  (via drill 0.35)
  Top 0.254: 109.12,66.62 110,66.62 RFV3.2 | 109.12,66.62 108.25,66.62 CFV3.2 | v54.75,50.25 54.84,50.34 STM32F303VB.25 | v71.75,71.38 v71.75,64 | 109.12,66.62 v109.12,71.38
  Bottom 0.254: v54.75,50.25 54.75,50.5 56.25,52 56.25,63.38 56.38,63.38 57,64 v71.75,64 | v109.12,71.38 v71.75,71.38

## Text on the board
tPlace: Designed in | North Wales | Made in UK
bPlace: Open Hardware
tNames: VT3 | SJ1 | VT2 | UART | 3.3 | 5V | RX | TX | DIO | CLK | RST | VT1 | MBUS
bNames: v0.2a | OpenEnergyMonitor | Development Board | emonSTM32
tDocu: 128.905 x / 105.791 y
